// generates a random noise signal, typical for disturbance signal. v1.2
// aParam explained
// Uniform 		: aParam[1] := min , aParam[2] := max limit
// Normal	 	: aParam[1] := mean, aParam[2] := standard deviation
// Exponential 	: aParam[1] := mean, aParam[2] := NA
// Gamma		: aParam[1] := deg. of freedom (max. 10), aParam[2] := NA (Gamma distribution: summing DOF number of exp. distributed variables)
// Chi-Squared 	: aParam[1] := mean, aParam[2] := standard deviation (Chi-squared (1DOF) is square of Gaussian Normal)
FUNCTION_BLOCK FB_NoiseGenerator
VAR_INPUT
	bEnable		: BOOL 	:= TRUE;	// set TRUE to generate the specified signal; set FALSE to reset the signal buffer
	nSeed		: INT	:= 1;	 	// seed value (initial value) for random function
	aParam		: ARRAY [1..2] OF LREAL := [0,1];	// specific parameter for chosen distribution type (see FB documentation)
	eDistrType	: E_DistributionType := E_DistributionType.Normal;
END_VAR
VAR_IN_OUT
	aSignal		: ARRAY[1..cOversamples] OF LREAL;
END_VAR
VAR_OUTPUT
	bError		: BOOL;
END_VAR

VAR
	bInit			: BOOL := TRUE;
	nInfiniteValue	: UDINT; // logarithm result is infinite probable caused by a random number of 0.

	nSamples		: UDINT; // array index
	fbRAND			: DRAND;

	// only for Gamma distribution
	nDof			: UINT; // array index
	nMaxDof 		: UINT;		
END_VAR
VAR CONSTANT
	cMaxDofGamma	: UINT := 10;
END_VAR

IF bEnable THEN
	IF bInit THEN
		// Flush out old data
		MEMSET(ADR(aSignal), 0, SIZEOF(aSignal));

		IF cOversamples > 0 THEN		
			fbRAND(Seed := nSeed); // initialize DRAND
			bInit := FALSE;
		ELSE
			bError := TRUE;
		END_IF
	END_IF
	
	// Enable function generator
	IF NOT bError THEN
		// random noise: typical for disturbance signal
		Rand();					
	END_IF
ELSE
	// Flush out old data
	MEMSET(ADR(aSignal), 0, SIZEOF(aSignal));
	
	bInit := TRUE;
	bError := FALSE;
END_IF

METHOD PRIVATE Rand
VAR_INPUT
END_VAR

VAR	
	fX1		: LREAL;
	fX2		: LREAL;
	fY1		: LREAL;
	fLnX1	: LREAL;
	fLength : LREAL;
	fD		: LREAL;
END_VAR
{warning disable C0371}

CASE eDistrType OF	
	E_DistributionType.Uniform:	
		fLength := aParam[2] - aParam[1];
		FOR nSamples := 1 TO cOversamples DO
			fbRAND(Num => fX1);	
			aSignal[nSamples] := fX1 * fLength + aParam[1];
		END_FOR
		
	E_DistributionType.Exponential:		
		FOR nSamples := 1 TO cOversamples DO
			fbRAND(Num => fX1);
			IF fX1 = 0 THEN
				fbRAND(Num => fX1);
			END_IF
			fLnX1 := LN(fX1);
			IF LrealIsFinite(fLnX1) THEN			
				aSignal[nSamples] := -aParam[1] * fLnX1;
			ELSE
				nInfiniteValue := nInfiniteValue + 1;
				aSignal[nSamples] := aParam[1];
			END_IF		
		END_FOR
		
	E_DistributionType.Normal:	
		FOR nSamples := 1 TO cOversamples DO
			// create 2 uniform distributed variables
			fbRAND(Num => fX1);
			IF fX1 = 0 THEN
				fbRAND(Num => fX1);
			END_IF		
			fbRAND(Num => fX2);
			IF fX2 = 0 THEN
				fbRAND(Num => fX2);
			END_IF	
			// create normal distribution
			fLnX1 := LN(fX1);
			IF LrealIsFinite(fLnX1) THEN			
				IF (fLnX1 < 0) THEN
					// Box Müller method
					fY1 := SQRT(-2*fLnX1)*COS(2*PI*fX2);
//					fY2 := SQRT(-2*LN(fX1))*SIN(2*PI*fX2);	
				END_IF
				aSignal[nSamples] := aParam[1] + aParam[2]*fY1;
			ELSE
				nInfiniteValue := nInfiniteValue + 1;
				aSignal[nSamples] := aParam[1];
			END_IF
		END_FOR	
	
	E_DistributionType.Gamma:		
		IF LREAL_TO_UINT(aParam[1]) > cMaxDofGamma THEN
			nMaxDof := cMaxDofGamma;
		ELSE
			nMaxDof := LREAL_TO_UINT(aParam[1]);
		END_IF
		//		
		FOR nSamples := 1 TO cOversamples DO
			aSignal[nSamples] := 0;
			FOR nDof := 1 TO nMaxDof DO
				fbRAND(Num => fX1);
				IF fX1 = 0 THEN
					fbRAND(Num => fX1);
				END_IF
				fLnX1 := LN(fX1);
				IF LrealIsFinite(fLnX1) THEN
					aSignal[nSamples] := aSignal[nSamples] - fLnX1;
				ELSE
					nInfiniteValue := nInfiniteValue + 1;
				END_IF		
			END_FOR	
		END_FOR

	//  1DOF: square of a single gaussian normal variable
	E_DistributionType.Chi_squared:
		FOR nSamples := 1 TO cOversamples DO
			// create 2 uniform distributed variables
			fbRAND(Num => fX1);
			IF fX1 = 0 THEN
				fbRAND(Num => fX1);
			END_IF	
			fbRAND(Num => fX2);
			IF fX2 = 0 THEN
				fbRAND(Num => fX2);
			END_IF	
			// create normal distribution
			fLnX1 := LN(fX1);
			IF LrealIsFinite(fLnX1) THEN				
				IF (fLnX1 < 0) THEN
					// Box Müller method
					fY1 := SQRT(-2*fLnX1)*COS(2*PI*fX2);
//					fY2 := SQRT(-2*LN(fX1))*SIN(2*PI*fX2);	
				END_IF	
				fD := aParam[1] + aParam[2]*fY1;
			ELSE
				nInfiniteValue := nInfiniteValue + 1;
				fD := aParam[1];		
			END_IF
			aSignal[nSamples] := fD * fD;
		END_FOR
		
END_CASE

{warning restore C0371}
END_METHOD

END_FUNCTION_BLOCK
